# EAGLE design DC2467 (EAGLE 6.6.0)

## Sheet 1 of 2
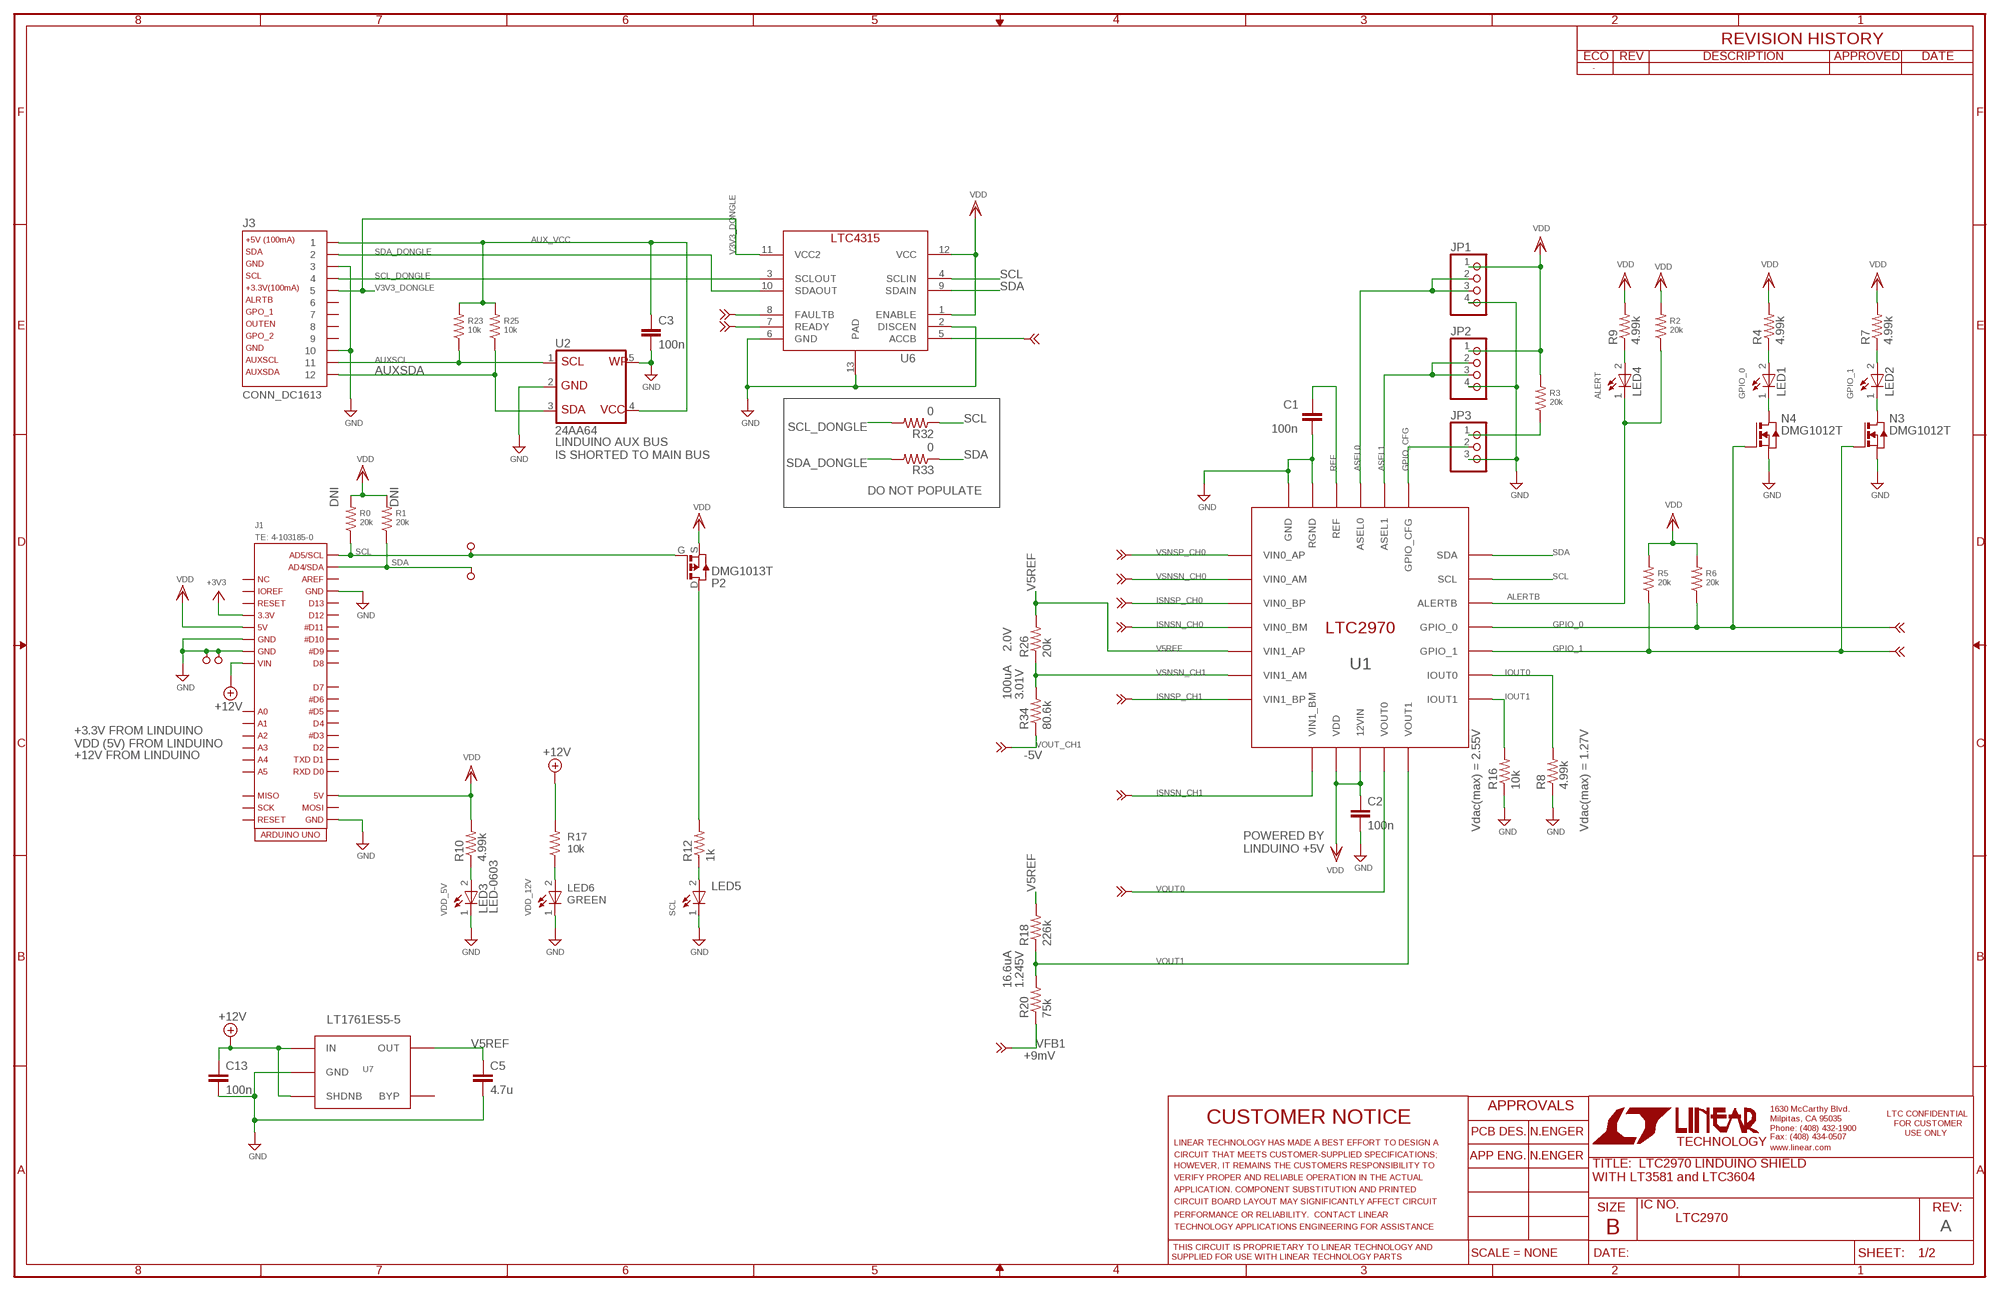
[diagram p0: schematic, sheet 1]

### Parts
C1  100n  CC0603_BOX  [C0603_BOX]
C2  100n  CC0603_BOX  [C0603_BOX]
C3  100n  CC0603_BOX  [C0603_BOX]
C5  4.7u  CC0603_BOX  [C0603_BOX]
C13  100n  CC0603_BOX  [C0603_BOX]
J1  TE: 4-103185-0  ARDUINO_UNO_MINI_SHIELD_SPIFL  [ADRUINO_UNO_STD_SHIELD_SPI]
J3  CONN_DC1613  [CONN_DC1613]
JP1  PINHD-1X4  [1X04]
JP2  PINHD-1X4  [1X04]
JP3  PINHD-1X3  [1X03]
LED1  LED-0603  [CHIPLED_0603]
LED2  LED-0603  [CHIPLED_0603]
LED3  LED-0603  [CHIPLED_0603]
LED4  LED-0603  [CHIPLED_0603]
LED5  LED-0603  [CHIPLED_0603]
LED6  GREEN  LED-0603  [CHIPLED_0603]
N3  DMG1012T  [SOT523-3]
N4  DMG1012T  [SOT523-3]
P2  DMG1013T  [SOT523-3]
R0  20k  RR0603_BOX  [R0603_BOX]
R1  20k  RR0603_BOX  [R0603_BOX]
R2  20k  RR0603_BOX  [R0603_BOX]
R3  20k  RR0603_BOX  [R0603_BOX]
R4  4.99k  RR0603_BOX  [R0603_BOX]
R5  20k  RR0603_BOX  [R0603_BOX]
R6  20k  RR0603_BOX  [R0603_BOX]
R7  4.99k  RR0603_BOX  [R0603_BOX]
R8  4.99k  RR0603_BOX  [R0603_BOX]
R9  4.99k  RR0603_BOX  [R0603_BOX]
R10  4.99k  RR0603_BOX  [R0603_BOX]
R12  1k  RR0603_BOX  [R0603_BOX]
R16  10k  RR0603_BOX  [R0603_BOX]
R17  10k  RR0603_BOX  [R0603_BOX]
R18  226k  RR0603_BOX  [R0603_BOX]
R20  75k  RR0603_BOX  [R0603_BOX]
R23  10k  RR0603_BOX  [R0603_BOX]
R25  10k  RR0603_BOX  [R0603_BOX]
R26  20k  RR0603_BOX  [R0603_BOX]
R32  0  RR0603_BOX  [R0603_BOX]
R33  0  RR0603_BOX  [R0603_BOX]
R34  80.6k  RR0603_BOX  [R0603_BOX]
TP1  TESPOINT_SMDSMD  [TESPOINT_SMD]
TP3  TESPOINT_SMDSMD  [TESPOINT_SMD]
TP4  TESTPOINT_BIG  [TP1]
TP5  TURRET_SMALL_2308TP  [TURRET_SMALL_2308]
TP6  TURRET_SMALL_2308TP  [TURRET_SMALL_2308]
TP7  TURRET_SMALL_2308TP  [TURRET_SMALL_2308]
TP10  TESPOINT_SMDSMD  [TESPOINT_SMD]
U1  LTC2970  [QFN-24]
U2  24AA64  [SOT-23-5]
U6  LTC4315  [DFN-12]
U7  LT1761ES5-5  [TSOT23-5]
U$1  FRAME_DC2467  [FRAME_DC2467]

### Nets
+3V3: J1.3V3
+12V: C13.1 J1.VIN R17.2 U7.P$1(IN) U7.P$3(SHDNB) ; also sheet 2
ALERTB: LED4.C R2.1 U1.P$17(ALERTB)
ASEL0: JP1.2 JP1.3 U1.P$22(ASEL0)
ASEL1: JP2.2 JP2.3 U1.P$21(ASEL1)
AUX_VCC: C3.1 J3.1 R23.2 R25.2 U2.4
AUXSCL: J3.11 R23.1 U2.1
AUXSDA: J3.12 R25.1 U2.3
GND: C1.2 C2.2 C3.2 C5.2 C13.2 J1.GND1 J1.GND2 J1.GND3 J1.GND4 J3.3 J3.10 JP1.4 JP2.4 JP3.3 LED3.C LED5.C LED6.C N3.S N4.S R8.1 R16.1 TP4.TP TP5.TP1 U1.P$24(RGND) U1.P$25(GND) U2.2 U2.5 U6.2(DISCEN) U6.6(GND) U6.13(PAD) U7.P$2(GND) ; also sheet 2
GPIO_0: N4.G R6.1 U1.P$16(GPIO_0) ; also sheet 2
GPIO_1: N3.G R5.1 U1.P$15(GPIO_1) ; also sheet 2
GPIO_CFG: JP3.2 U1.P$20(GPIO_CFG)
IOUT0: R8.2 U1.P$14(IOUT0)
IOUT1: R16.2 U1.P$13(IOUT1)
ISNSN_CH0: U1.P$4(VIN0_BM) ; also sheet 2
ISNSN_CH1: U1.P$8(VIN1_BM) ; also sheet 2
ISNSP_CH0: U1.P$3(VIN0_BP) ; also sheet 2
ISNSP_CH1: U1.P$7(VIN1_BP) ; also sheet 2
N$1: LED1.C N4.D
N$2: LED1.A R4.1
N$3: LED2.C N3.D
N$4: LED2.A R7.1
N$6: LED3.A R10.1
N$7: LED4.A R9.1
N$9: LED5.A R12.1
N$10: P2.D R12.2
N$11: LED6.A R17.1
N$16: JP3.1 R3.1
N$26: TP3.P$1 U6.8(FAULTB)
N$29: TP10.P$1 U6.7(READY)
N$30: TP1.P$1 U6.5(ACCB)
REF: C1.1 U1.P$23(REF)
SCL: J1.SCL P2.G R0.1 R32.1 TP7.TP1 U1.P$18(SCL) U6.4(SCLIN)
SCL_DONGLE: J3.4 R32.2 U6.3(SCLOUT)
SDA: J1.SDA R1.1 R33.1 TP6.TP1 U1.P$19(SDA) U6.9(SDAIN)
SDA_DONGLE: J3.2 R33.2 U6.10(SDAOUT)
V3V3_DONGLE: J3.5 U6.11(VCC2)
V5REF: C5.1 R18.2 R26.2 U1.P$5(VIN1_AP) U7.P$5(OUT)
VDD: C2.1 J1.5V J1.5V1 JP1.1 JP2.1 P2.S R0.2 R1.2 R2.2 R3.2 R4.2 R5.2 R6.2 R7.2 R9.2 R10.2 U1.P$9(VDD) U1.P$10(12VIN) U6.1(ENABLE) U6.12(VCC)
VFB1: R20.1 ; also sheet 2
VOUT0: U1.P$11(VOUT0) ; also sheet 2
VOUT1: R18.1 R20.2 U1.P$12(VOUT1)
VOUT_CH1: R34.1 ; also sheet 2
VSNSN_CH0: U1.P$2(VIN0_AM) ; also sheet 2
VSNSN_CH1: R26.1 R34.2 U1.P$6(VIN1_AM)
VSNSP_CH0: U1.P$1(VIN0_AP) ; also sheet 2
Unconnected: J1.A0 J1.A1 J1.A2 J1.A3 J1.A4 J1.A5 J1.D0 J1.D1 J1.D2 J1.D3 J1.D4 J1.D5 J1.D6 J1.D7 J1.D8 J1.D9 J1.D10 J1.D11 J1.D12 J1.D13 J1.MISO J1.MOSI J1.NC J1.REF J1.RST1 J1.RST2 J1.SCK J1.VIO J3.6 J3.7 J3.8 J3.9 U7.P$4(BYP)

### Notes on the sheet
- ALERT | GPIO_0 | GPIO_1
- LINDUINO AUX BUS 
  IS SHORTED TO MAIN BUS
- DO NOT POPULATE
- DNI | DNI
- 2.0V
- 100uA | 3.01V
- +3.3V FROM LINDUINO
  VDD (5V) FROM LINDUINO
- +12V FROM LINDUINO | -5V
- POWERED BY
  LINDUINO +5V
- Vdac(max) = 2.55V | Vdac(max) = 1.27V
- VDD_5V | VDD_12V | SCL
- 16.6uA | 1.245V
- LT1761ES5-5
- +9mV
- A

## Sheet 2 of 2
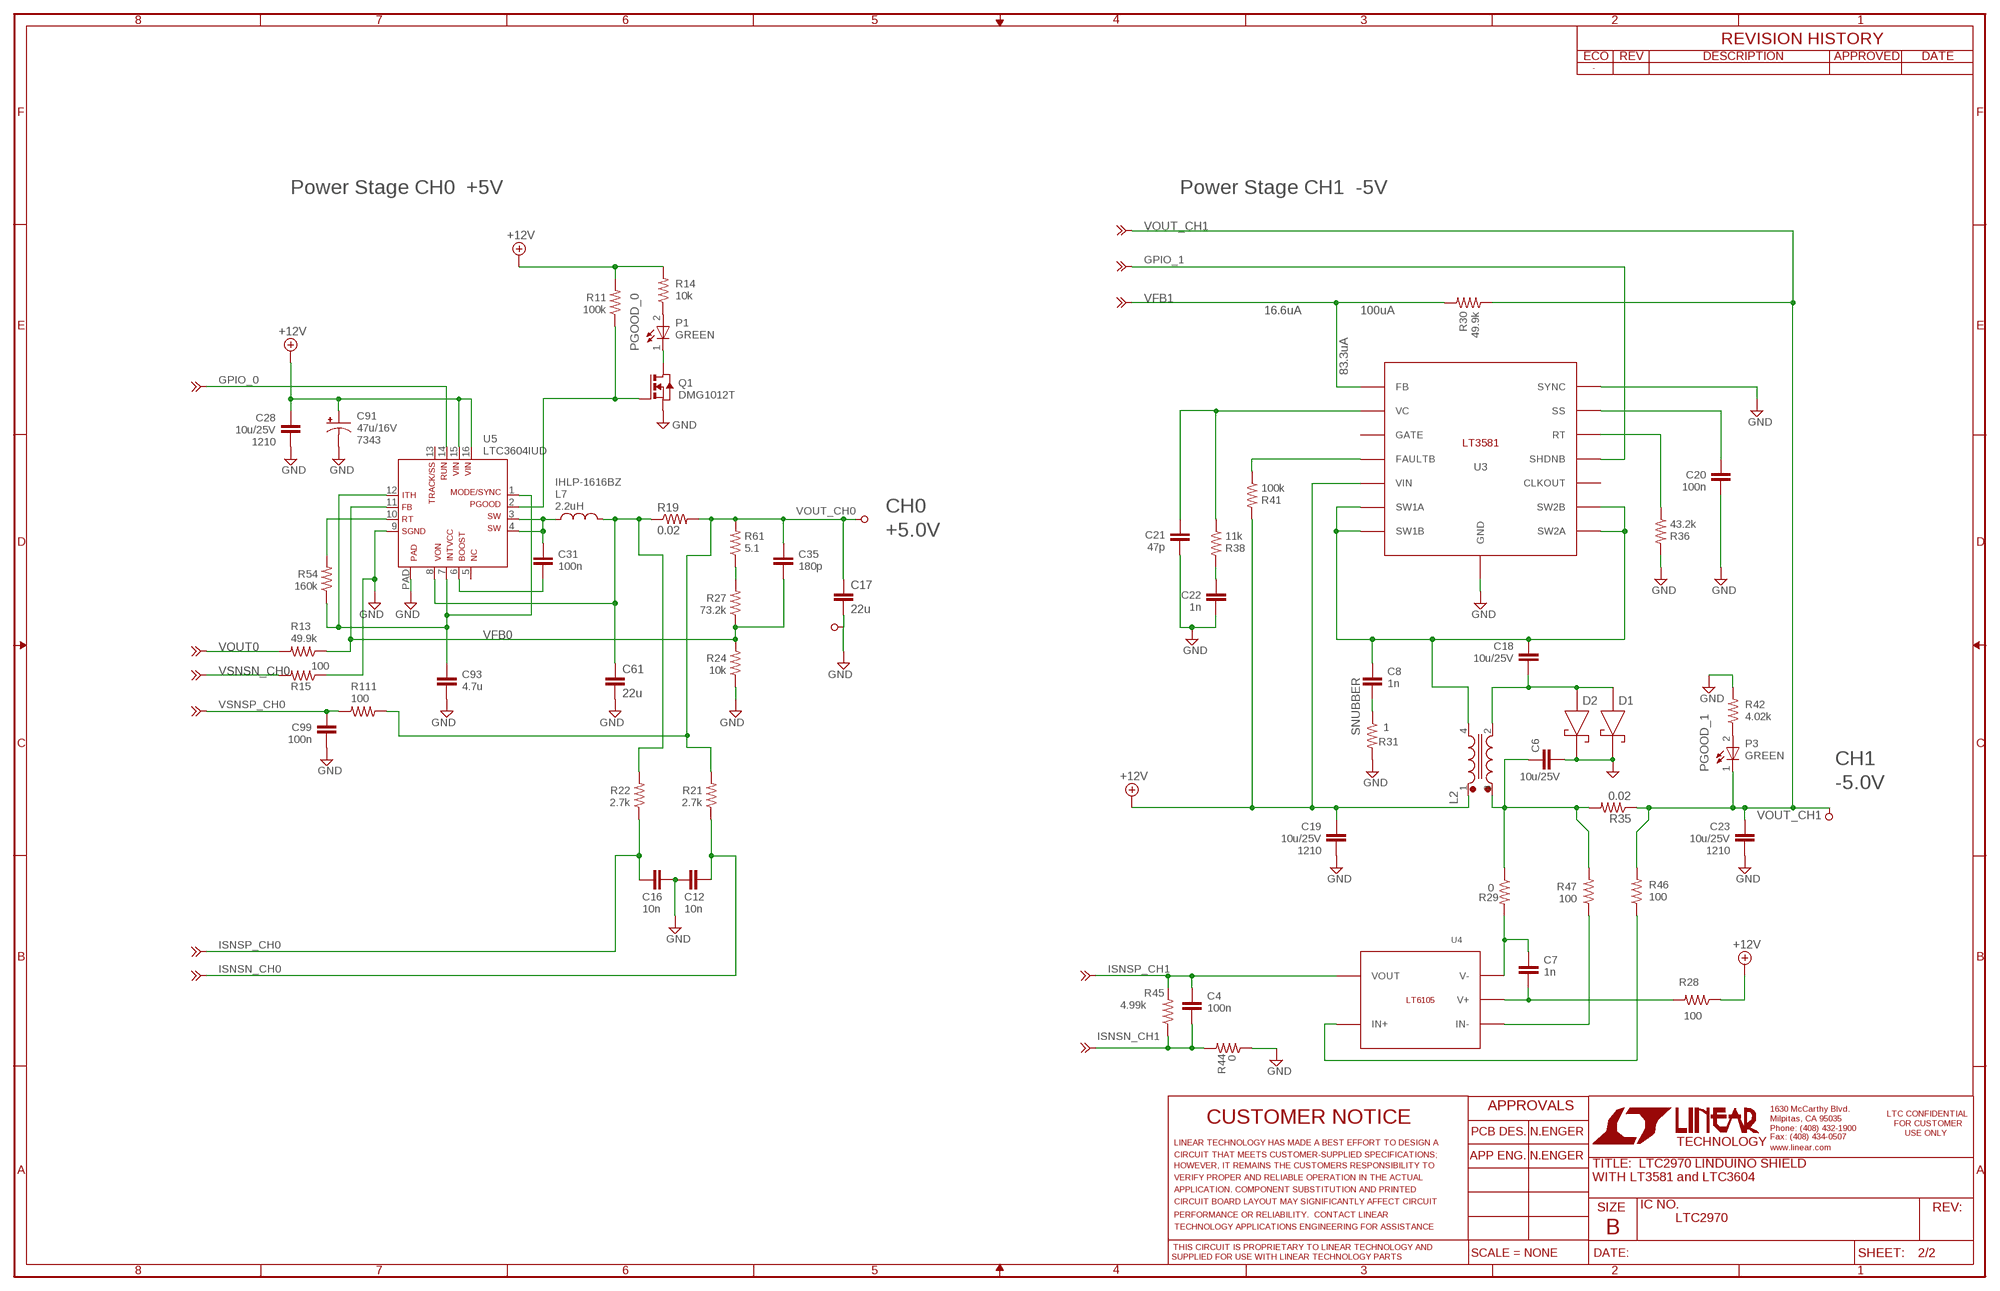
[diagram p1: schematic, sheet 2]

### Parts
C4  100n  CC0603_BOX  [C0603_BOX]
C6  10u/25V  CC1210_BOX  [C1210_BOX]
C7  1n  CC0603_BOX  [C0603_BOX]
C8  1n  CC0603_BOX  [C0603_BOX]
C12  10n  CC0603_BOX  [C0603_BOX]
C16  10n  CC0603_BOX  [C0603_BOX]
C17  22u  CC1210_BOX  [C1210_BOX]
C18  10u/25V  CC1210_BOX  [C1210_BOX]
C19  10u/25V  CC1210_BOX  [C1210_BOX]
C20  100n  CC0603_BOX  [C0603_BOX]
C21  47p  CC0603_BOX  [C0603_BOX]
C22  1n  CC0603_BOX  [C0603_BOX]
C23  10u/25V  CC1210_BOX  [C1210_BOX]
C28  10u/25V  CC1210_BOX  [C1210_BOX]
C31  100n  CC0603_BOX  [C0603_BOX]
C35  180p  CC0603_BOX  [C0603_BOX]
C61  22u  CC1210_BOX  [C1210_BOX]
C91  47u/16V  CPOL-USCT7343  [CT7343]
C93  4.7u  CC0603_BOX  [C0603_BOX]
C99  100n  CC0603_BOX  [C0603_BOX]
D1  DFLS220L  [POWERDI-123]
D2  DFLS220L  [POWERDI-123]
L2  WE-TDC_8038  [WE-TDC_80XX]
L7  2.2uH  LVISHAY-IHLP1616AB  [IHLP_1616AB]
P1  GREEN  LED-0603  [CHIPLED_0603]
P3  GREEN  LED-0603  [CHIPLED_0603]
Q1  DMG1012T  [SOT523-3]
R11  100k  RR0603_BOX  [R0603_BOX]
R13  49.9k  RR0603_BOX  [R0603_BOX]
R14  10k  RR0603_BOX  [R0603_BOX]
R15  100  RR0603_BOX  [R0603_BOX]
R19  0.02  RR1210  [R1210]
R21  2.7k  RR0603_BOX  [R0603_BOX]
R22  2.7k  RR0603_BOX  [R0603_BOX]
R24  10k  RR0603_BOX  [R0603_BOX]
R27  73.2k  RR0603_BOX  [R0603_BOX]
R28  100  RR0603_BOX  [R0603_BOX]
R29  0  RR0603_BOX  [R0603_BOX]
R30  49.9k  RR0603_BOX  [R0603_BOX]
R31  1  RR0603_BOX  [R0603_BOX]
R35  0.02  RR1210  [R1210]
R36  43.2k  RR0603_BOX  [R0603_BOX]
R38  11k  RR0603_BOX  [R0603_BOX]
R41  100k  RR0603_BOX  [R0603_BOX]
R42  4.02k  RR0603_BOX  [R0603_BOX]
R44  0  RR0603_BOX  [R0603_BOX]
R45  4.99k  RR0603_BOX  [R0603_BOX]
R46  100  RR0603_BOX  [R0603_BOX]
R47  100  RR0603_BOX  [R0603_BOX]
R54  160k  RR0603_BOX  [R0603_BOX]
R61  5.1  RR0603_BOX  [R0603_BOX]
R111  100  RR0603_BOX  [R0603_BOX]
TP2  TESTPOINT_BIG  [TP1]
TP8  TESTPOINT_BIG  [TP1]
TP9  TESTPOINT_BIG  [TP1]
U3  LT3581  [DFN-14]
U4  LT6105  [DFN-6]
U5  LTC3604IUD  [QFN16_3X3]
U$3  FRAME_DC2467  [FRAME_DC2467]
VSNSN1  TESPOINT_SMD  TESPOINT_SMDVIA  [VIA]
VSNSN2  TESPOINT_SMD  TESPOINT_SMDVIA  [VIA]
VSNSN3  TESPOINT_SMD  TESPOINT_SMDVIA  [VIA]
VSNSN4  TESPOINT_SMD  TESPOINT_SMDVIA  [VIA]
VSNSN11  TESPOINT_SMD  TESPOINT_SMDVIA  [VIA]
VSNSN56  TESPOINT_SMD  TESPOINT_SMDVIA  [VIA]
VSNSN57  TESPOINT_SMD  TESPOINT_SMDVIA  [VIA]
VSNSN58  TESPOINT_SMD  TESPOINT_SMDVIA  [VIA]
VSNSN59  TESPOINT_SMD  TESPOINT_SMDVIA  [VIA]

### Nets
+12V: C19.2 C28.2 C91.+ L2.1 R11.2 R14.2 R28.1 R41.2 U3.P$5(VIN) U5.15 U5.16 ; also sheet 1
GND: C6.1 C12.2 C16.1 C17.2 C19.1 C20.1 C21.1 C22.1 C23.1 C28.1 C61.2 C91.- C93.2 C99.1 D1.P$1 D2.P$1 Q1.S R15.1 R24.1 R31.2 R36.2 R42.2 R44.1 TP9.TP U3.P$14(SYNC) U3.P$15(GND) U5.9 U5.PAD ; also sheet 1
GPIO_0: U5.14 VSNSN11.1 ; also sheet 1
GPIO_1: U3.P$11(SHDNB) VSNSN2.1 ; also sheet 1
INTVCC_LTC3604: C93.1 R54.1 U5.1 U5.7 U5.12
ISNSN_CH0: C12.1 R21.1 VSNSN56.1 ; also sheet 1
ISNSN_CH1: C4.1 R44.2 R45.1 ; also sheet 1
ISNSP_CH0: C16.2 R22.1 VSNSN57.1 ; also sheet 1
ISNSP_CH1: C4.2 R45.2 U4.P$4(VOUT) VSNSN4.1 ; also sheet 1
N$5: R47.1 U4.P$1(IN-)
N$8: R27.2 R61.1
N$12: C7.2 R29.2 U4.P$3(V-) U4.P$9(V-)
N$13: C7.1 R28.2 U4.P$2(V+)
N$14: C8.1 R31.1
N$15: C18.1 D1.P$2 D2.P$2 L2.2
N$18: C8.2 C18.2 L2.4 U3.P$6(SW1A) U3.P$7(SW1B) U3.P$8(SW2A) U3.P$9(SW2B)
N$19: P1.A R14.1
N$20: P1.C Q1.D
N$21: R41.1 U3.P$4(FAULTB)
N$22: R36.1 U3.P$12(RT)
N$23: C20.2 U3.P$13(SS)
N$25: Q1.G R11.1 U5.2
N$27: C6.2 L2.3 R29.1 R35.2 R47.2
N$28: P3.A R42.1
N$31: C22.2 R38.2
N$32: C21.2 R38.1 U3.P$2(VC)
N$33: R46.1 U4.P$6(IN+)
N$70: C31.2 U5.6
N$78: R54.2 U5.10
SW1: C31.1 L7.1 U5.3 U5.4
V1: C61.1 L7.2 R19.1 R22.2 U5.8
VFB0: C35.2 R13.1 R24.2 R27.1 U5.11
VFB1: R30.2 U3.P$1(FB) VSNSN3.1 ; also sheet 1
VOUT0: R13.2 VSNSN58.1 ; also sheet 1
VOUT_CH0: C17.1 C35.1 R19.2 R21.2 R61.2 R111.1 TP8.TP
VOUT_CH1: C23.2 P3.C R30.1 R35.1 R46.2 TP2.TP ; also sheet 1
VSNSN_CH0: R15.2 VSNSN1.1 ; also sheet 1
VSNSP_CH0: C99.2 R111.2 VSNSN59.1 ; also sheet 1
Unconnected: U3.P$3(GATE) U3.P$10(CLKOUT) U5.5 U5.13

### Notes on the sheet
- Power Stage CH0  +5V | Power Stage CH1  -5V
- 16.6uA | 100uA
- PGOOD_0
- 83.3uA
- 1210
- 7343
- IHLP-1616BZ
- CH0
- +5.0V
- SNUBBER
- CH1
- PGOOD_1
- -5.0V
- 1210 | 1210

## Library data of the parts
C1-C8 C12 C13 C16-C23 C28 C31 C35 C61 C93 C99 = kalin:C: CAPACITOR, European symbol
C91 = rcl:CPOL-US: POLARIZED CAPACITOR, American symbol
D1 D2 = nengerLib:DFLS220L: DIODES INC DFLS220L
J1 = FOO:ARDUINO_UNO_MINI_SHIELD_SPI: Arduino UNO Mini Shield With SPI
J3 = kalin:CONN_DC1613: Connector for LT DC1613 USB Dongle
JP1 JP2 = LIBSnengerLib:PINHD-1X4: PIN HEADER
JP3 = LIBSnengerLib:PINHD-1X3: PIN HEADER
L2 = Wurth_Elektronik_Passive_rev15f:WE-TDC: SEPIC SMD Coupled Inductor Characteristics Core material: NiZn Low profile Magnetical shielded which results in a low leakage field 8x8 mm case 1:1 transformer Low self-losses High self resonance frequency Coupled inductor with two identical windings Operating temperature: –40 °C up to +125 °C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
L7 = kalin:L: Inductor
LED1-LED6 P1 P3 = kalin:LED-0603: SMD LED in R0603
N3 N4 Q1 = nengerLib:DMG1012T: Diodes Inc. N-Channel Enhancement Mode N-MOSFET
P2 = FOO:DMG1013T: Diodes Inc. P-Channel Enhancement Mode P-MOSFET
R0 R1-R36 R38 R41 R42 R44-R47 R54 R61 R111 = kalin:R: RESISTOR, American symbol
TP1 TP3 TP10 VSNSN1-VSNSN4 VSNSN11 VSNSN56-VSNSN59 = kalin:TESPOINT_SMD: SMALL SMD Test Point
TP2 TP4 TP8 TP9 = kalin:TESTPOINT_BIG: Large Test Point
TP5-TP7 = kalin:TURRET_SMALL_2308: Small Test Turret Mill-Max 2308
U1 = LTC-DEVICES:LTC2970: LTC2970 Dual I2C Power Supply Monitor and Margining Controller
U2 = kalin:24AA64: 64K I2C? Serial EEPROM
U3 = LTC-DEVICES:LT3581: LT3581 3.3A Boost/Inverting DC/DC Converter with Fault Protection
U4 = LTC-DEVICES:LT6105
U5 = kalin:LTC3604: 2.5A, 15V Monolithic Synchronous Step-Down Regulator
U6 = LTC-DEVICES:LTC4315: 2-Wire Bus Buffer with High Noise Margin
U7 = nengerLib:LT1761ES5-5
U$1 U$3 = nengerFramesLib:FRAME_DC2467

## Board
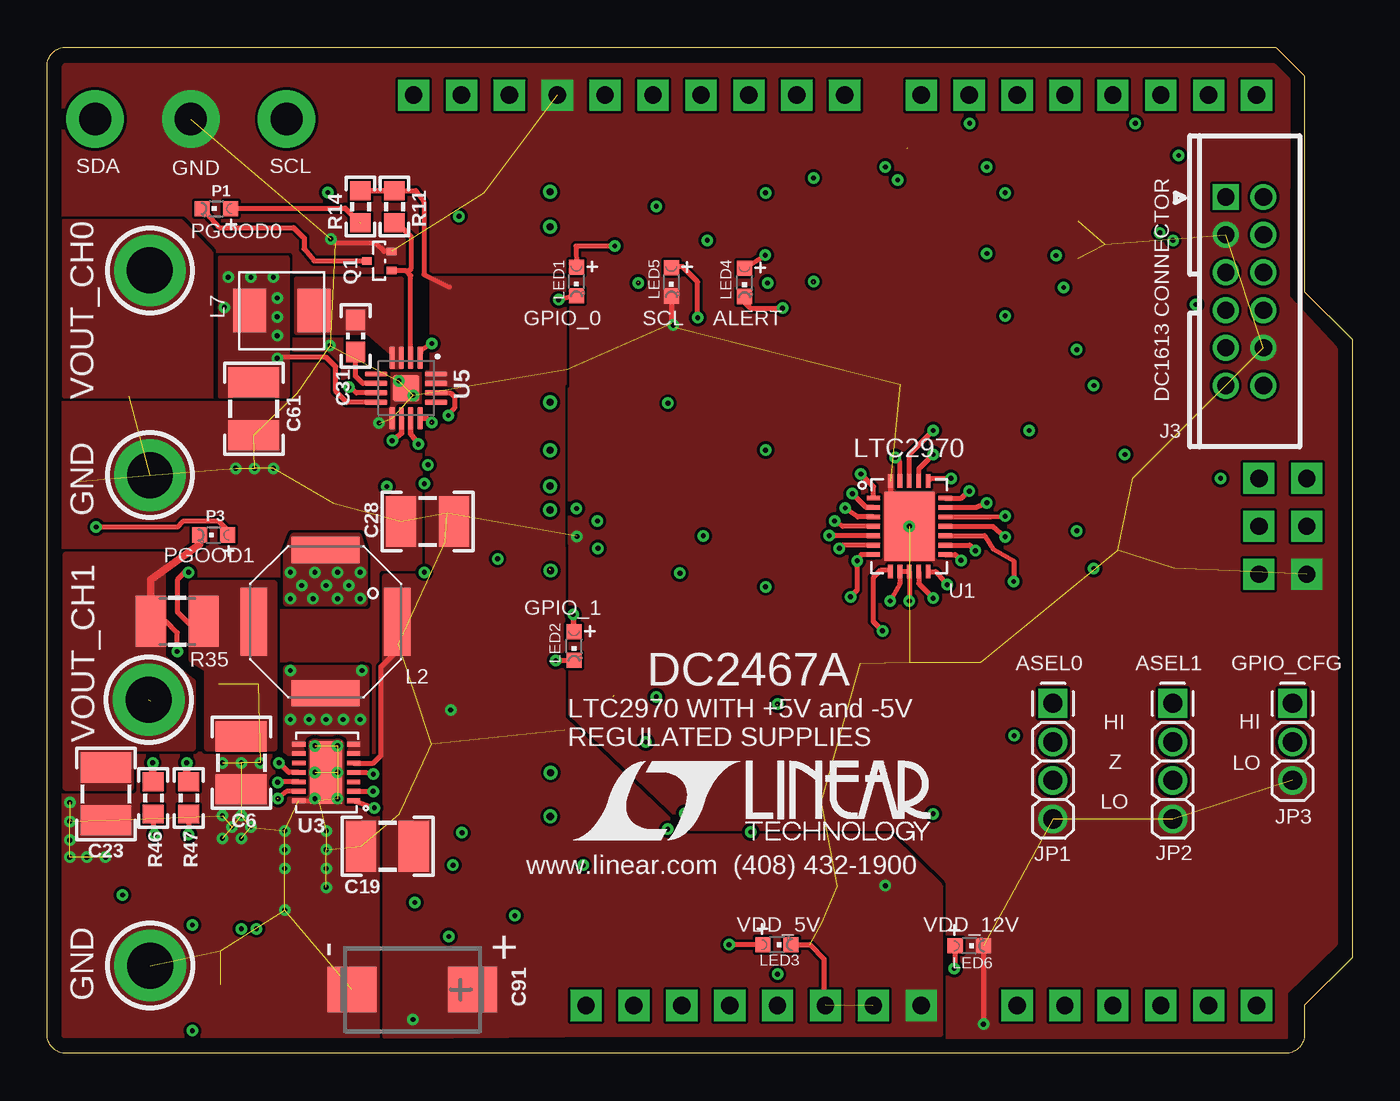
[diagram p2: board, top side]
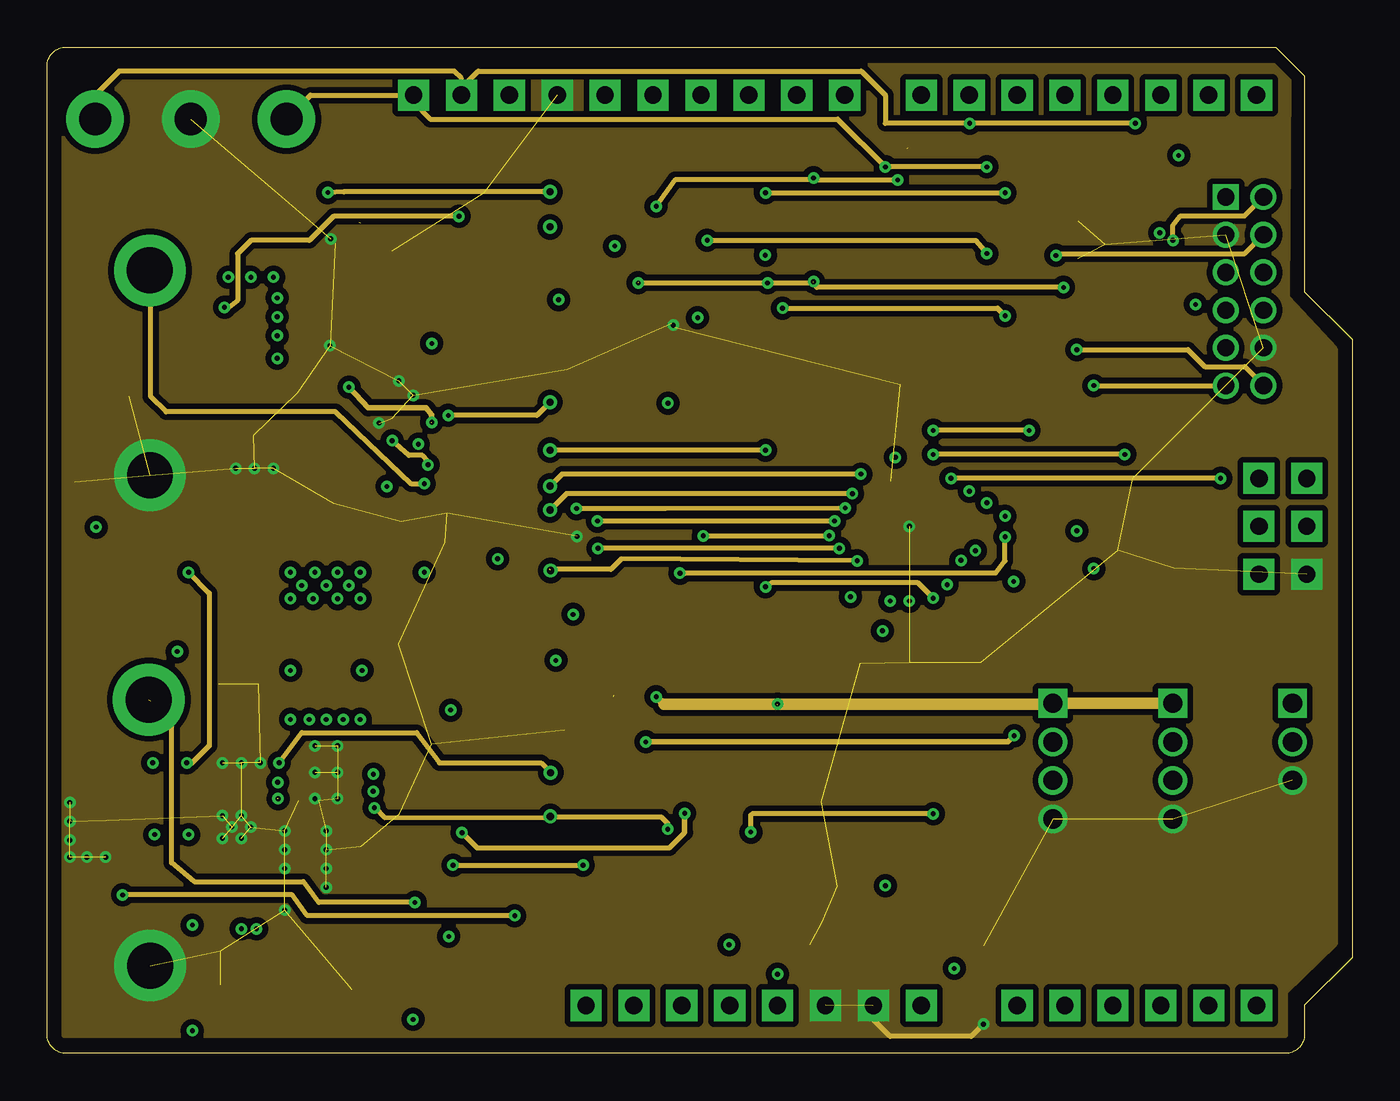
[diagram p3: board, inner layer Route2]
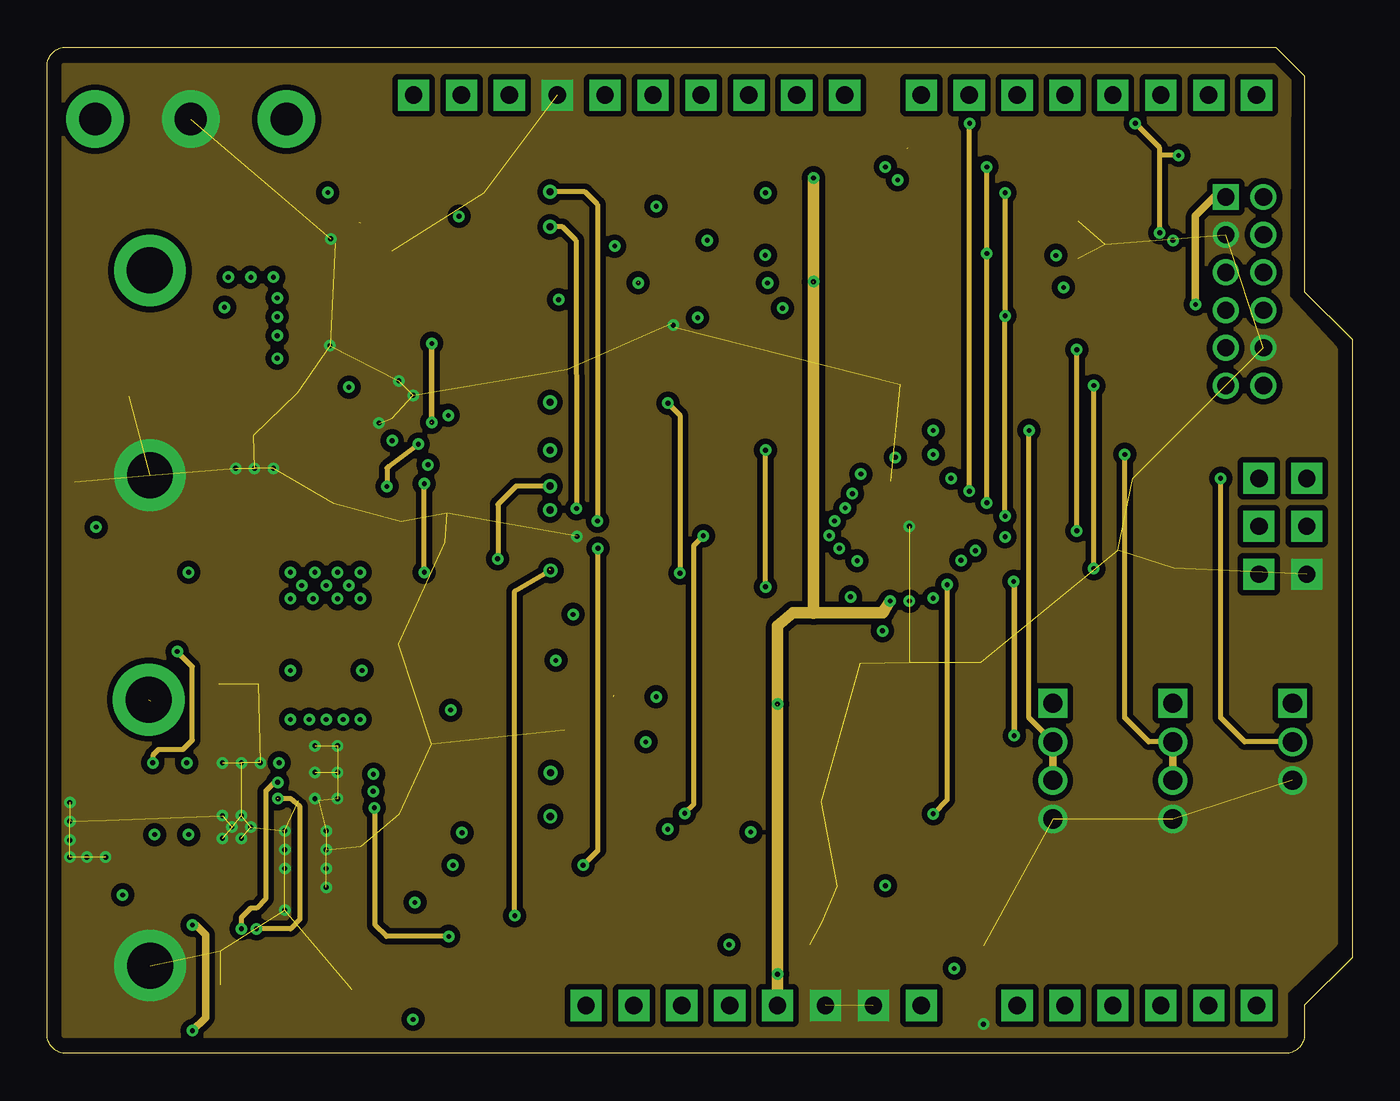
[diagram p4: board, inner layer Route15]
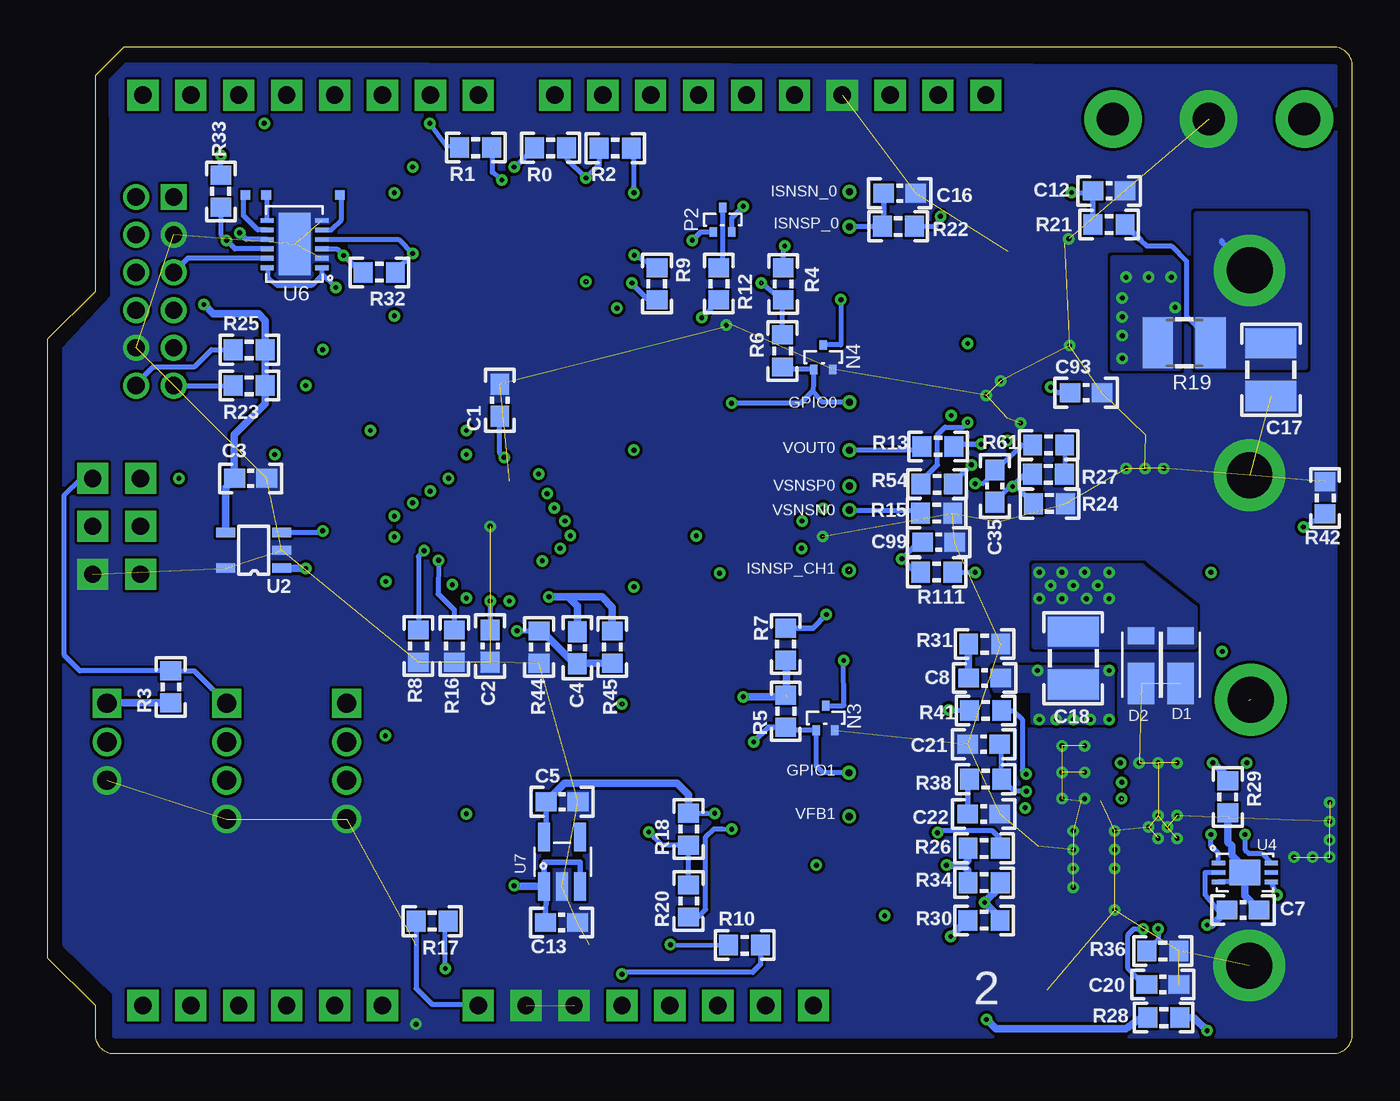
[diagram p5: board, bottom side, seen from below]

Size 69.22 x 53.34 mm. Coordinates in mm from the lower left corner, seen from the top.
Copper layers (1+2*15+16): Top 0.07mm / dielectric 0.23mm / Route2 0.035mm / dielectric 1.01mm / Route15 0.035mm / dielectric 0.2mm / Bottom 0.07mm
Design rules "nicks-panel": minimum track width 6mil, minimum drill 10mil, track to track 6mil, track to pad 6mil, pad to pad 6mil, via to via 6mil, smd to smd 6mil, copper to edge 20mil, drill to drill 8mil, minimum pad ring 7mil, minimum via ring 7mil, stop-mask expansion 2.5mil, vias tented up to drill 14mil, thermal gap 10mil

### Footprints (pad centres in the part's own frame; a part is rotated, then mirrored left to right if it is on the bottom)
C0603_BOX = smd 1.1 x 1: 1 -0.85,0; 2 0.85,0
C1210_BOX = smd 1.6 x 2.7: 1 -1.4,0; 2 1.4,0
CT7343 = smd 2.6 x 2.4: + -3.2,0; - 3.2,0
POWERDI-123 = smd 2.2 x 1.4: P$1 -1.6,0 | smd 0.9 x 1.4: P$2 0.95,0
ADRUINO_UNO_STD_SHIELD_SPI = drill 0.914 pad 1.651 square: 3V3 18.415,2.54; 5V 20.955,2.54; 5V1 49.022,30.48; A0 33.655,2.54; A1 36.195,2.54; A2 38.735,2.54; A3 41.275,2.54; A4 43.815,2.54; A5 46.355,2.54; D0 46.355,50.8; D1 43.815,50.8; D2 41.275,50.8; D3 38.735,50.8; D4 36.195,50.8; D5 33.655,50.8; D6 31.115,50.8; D7 28.575,50.8; D8 24.511,50.8; D9 21.971,50.8; D10 19.431,50.8; D11 16.891,50.8; D12 14.351,50.8; D13 11.811,50.8; GND1 23.495,2.54; GND2 26.035,2.54; GND3 9.271,50.8; GND4 49.022,25.4; MISO 46.482,30.48; MOSI 49.022,27.94; NC 10.795,2.54; REF 6.731,50.8; RST1 15.875,2.54; RST2 46.482,25.4; SCK 46.482,27.94; SCL 1.651,50.8; SDA 4.191,50.8; VIN 28.575,2.54; VIO 13.335,2.54
CONN_DC1613 = drill 0.914 square: 1 -5,-1 | drill 0.914: 2 -5,1; 3 -3,-1; 4 -3,1; 5 -1,-1; 6 -1,1; 7 1,-1; 8 1,1; 9 3,-1; 10 3,1; 11 5,-1; 12 5,1
1X04 = drill 1.016 square: 1 -2.05,0 | drill 1.016: 2 0,0; 3 2.04,0; 4 4.09,0
1X03 = drill 1.016 square: 1 -2.05,0 | drill 1.016: 2 0,0; 3 2.04,0
WE-TDC_80XX = smd 3.6 x 1.4: 1 0,3.8; 3 0,-3.8 | smd 1.4 x 3.6: 2 -3.8,0; 4 3.8,0
IHLP_1616AB = smd 1.75 x 2.3: 1 -1.7,0; 2 1.7,0
CHIPLED_0603 = smd 0.8 x 0.8: A 0,-0.75; C 0,0.75
SOT523-3 = smd 0.4 x 0.51: D 0,0.65; G -0.5,-0.65; S 0.5,-0.65
R0603_BOX = smd 1 x 1.1: 1 -0.85,0; 2 0.85,0
R1210 = smd 1.6 x 2.7: 1 -1.4,0; 2 1.4,0
TESPOINT_SMD = smd 0.508 x 0.508: P$1 0,0
TP1 = drill 2.438 pad 3.81: TP 0,0
TURRET_SMALL_2308 = drill 1.702 pad 3.048: TP1 0,0
QFN-24 = smd 0.7 x 0.25: P$1 -1.9,1.5; P$2 -1.9,1; P$3 -1.9,0.5; P$4 -1.9,0; P$5 -1.9,-0.5; P$6 -1.9,-1; P$7 -1.9,-1.5; P$13 1.9,-1.5; P$14 1.9,-1; P$15 1.9,-0.5; P$16 1.9,0; P$17 1.9,0.5; P$18 1.9,1; P$19 1.9,1.5 | smd 0.25 x 0.7: P$8 -1,-2.4; P$9 -0.5,-2.4; P$10 0,-2.4; P$11 0.5,-2.4; P$12 1,-2.4; P$20 1,2.4; P$21 0.5,2.4; P$22 0,2.4; P$23 -0.5,2.4; P$24 -1,2.4 | smd 2.65 x 3.65: P$25 0,0
SOT-23-5 = smd 1 x 0.5: 1 -1.649,0.95; 2 -1.649,0; 3 -1.649,-0.95; 4 1.333,-0.95; 5 1.333,0.95
DFN-14 = smd 0.25 x 0.7: P$1 -1.5,-1.45; P$2 -1,-1.45; P$3 -0.5,-1.45; P$4 0,-1.45; P$5 0.5,-1.45; P$6 1,-1.45; P$7 1.5,-1.45; P$8 1.5,1.45; P$9 1,1.45; P$10 0.5,1.45; P$11 0,1.45; P$12 -0.5,1.45; P$13 -1,1.45; P$14 -1.5,1.45 | smd 3.3 x 1.7: P$15 0,0
DFN-6 = smd 0.25 x 0.7: P$1 -0.5,-1.4; P$2 0,-1.4; P$3 0.5,-1.4; P$4 0.5,1.4; P$5 0,1.4; P$6 -0.5,1.4 | smd 1.35 x 1.65: P$9 0,0
QFN16_3X3 = smd 1.2 x 0.3: 1 -1.711,0.734; 2 -1.711,0.234; 3 -1.711,-0.266; 4 -1.711,-0.766; 9 1.489,-0.766; 10 1.489,-0.266; 11 1.489,0.234; 12 1.489,0.734 | smd 0.3 x 1.2: 5 -0.861,-1.616; 6 -0.361,-1.616; 7 0.139,-1.616; 8 0.639,-1.616; 13 0.639,1.584; 14 0.139,1.584; 15 -0.361,1.584; 16 -0.861,1.584 | smd 1.4 x 1.4: PAD -0.111,-0.016
DFN-12 = smd 0.7 x 0.25: 1 -1.45,1.25; 2 -1.45,0.75; 3 -1.45,0.25; 4 -1.45,-0.25; 5 -1.45,-0.75; 6 -1.45,-1.25; 7 1.45,-1.25; 8 1.45,-0.75; 9 1.45,-0.25; 10 1.45,0.25; 11 1.45,0.75; 12 1.45,1.25 | smd 1.7 x 3.3: 13 0,0
TSOT23-5 = smd 0.63 x 1.5: P$1 -0.95,-1.31; P$2 0,-1.31; P$3 0.95,-1.31; P$4 0.95,1.31; P$5 -0.95,1.31
VIA = drill 0.381: 1 0,0

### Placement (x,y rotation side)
C1  45.21,34.62 90 bottom
C2  45.72,21.59 270 bottom
C3  58.42,30.48 0 bottom
C4  41.1,21.5 90 bottom
C5  41.91,13.34 0 bottom
C6  10.3,15.4 90 top
C7  5.8,7.6 0 bottom
C8  19.5,19.9 0 bottom
C12  12.9,45.72 0 bottom
C13  41.94,6.93 0 bottom
C16  24,45.59 180 bottom
C17  4.32,36.25 270 bottom
C18  14.8,20.95 270 bottom
C19  18.05,10.98 0 top
C20  10.05,3.65 180 bottom
C21  19.55,16.39 0 bottom
C22  19.55,12.69 180 bottom
C23  3.12,13.75 90 top
C28  20.18,28.19 0 top
C31  16.36,38.02 270 top
C35  18.96,30.07 270 bottom
C61  10.96,34.17 270 top
C91  19.37,3.38 180 top
C93  14.12,35.03 0 bottom
C99  21.94,27.1 180 bottom
D1  9.1,21.2 90 bottom
D2  11.2,21.2 90 bottom
DRILEGEND  [DRILEGEND]  not placed on the board
J1  17.78,0 0 top
J3  63.5,40.4 270 top
JP1  53.34,16.51 270 top
JP2  59.69,16.51 270 top
JP3  66.04,16.51 270 top
L2  14.77,22.89 270 top
L7  12.45,39.37 180 top
LED1  28.07,40.92 180 top
LED2  27.94,21.59 180 top
LED3  38.7,5.76 270 top
LED4  36.98,40.87 180 top
LED5  33.1,40.9 180 top
LED6  48.9,5.7 270 top
N3  27.94,17.78 0 bottom
N4  28.07,36.91 0 bottom
P1  8.98,44.78 90 top
P2  33.4,44.2 0 bottom
P3  8.83,27.48 90 top
Q1  17.61,42.01 90 top
R0  42.52,48.01 0 bottom
R1  46.49,48.02 0 bottom
R2  39.09,47.98 180 bottom
R3  62.66,19.43 90 bottom
R4  30.18,40.79 270 bottom
R5  30.05,18.14 90 bottom
R6  30.23,37.24 90 bottom
R7  30.05,21.69 270 bottom
R8  49.53,21.59 90 bottom
R9  36.88,40.8 270 bottom
R10  32.23,5.74 0 bottom
R11  18.42,44.88 90 top
R12  33.6,40.8 90 bottom
R13  21.97,32.17 180 bottom
R14  16.61,44.88 90 top
R15  22.05,28.63 180 bottom
R16  47.62,21.59 90 bottom
R17  48.8,7 180 bottom
R18  35.2,11.89 90 bottom
R19  8.92,37.67 0 bottom
R20  35.2,8.08 90 bottom
R21  12.9,43.94 0 bottom
R22  24.08,43.84 0 bottom
R23  58.5,35.4 0 bottom
R24  16.06,29.14 180 bottom
R25  58.5,37.3 0 bottom
R26  19.52,10.87 0 bottom
R27  16.12,30.71 0 bottom
R28  10,1.9 0 bottom
R29  6.6,13.6 270 bottom
R30  19.53,7.05 180 bottom
R31  19.5,21.7 0 bottom
R32  51.6,41.4 180 bottom
R33  60,45.7 270 bottom
R34  19.52,9.04 180 bottom
R35  6.9,22.9 0 top
R36  10.05,5.43 0 bottom
R38  19.45,14.53 180 bottom
R41  19.45,18.17 180 bottom
R42  1.45,29.45 90 bottom
R44  43.13,21.54 90 bottom
R45  39.25,21.54 90 bottom
R46  5.63,13.54 90 top
R47  7.51,13.54 90 top
R54  22.02,30.18 0 bottom
R61  16.11,32.25 180 bottom
R111  22.04,25.5 180 bottom
TP1  53.7,45.5 0 bottom
TP2  5.39,18.75 270 top
TP3  58.7,45.5 0 bottom
TP4  5.46,4.66 0 top
TP5  7.62,49.53 0 top
TP6  2.54,49.53 0 top
TP7  12.7,49.53 0 top
TP8  5.45,41.5 270 top
TP9  5.45,30.66 270 top
TP10  57.6,45.5 0 bottom
U1  45.72,27.94 0 top
U2  58.42,26.67 180 bottom
U3  14.8,14.89 90 top
U4  5.7,9.59 270 bottom
U5  19.05,35.15 270 top
U6  56.1,42.9 180 bottom
U7  41.91,10.16 0 bottom
U$1  not placed on the board
U$3  not placed on the board
U$6  [LT_LOGO_LARGE]  27.8,11.2 0 top
VSNSN1  26.67,28.8 270 top
VSNSN2  26.7,14.88 90 top
VSNSN3  26.68,12.56 0 top
VSNSN4  26.7,25.6 0 top
VSNSN11  26.67,34.52 270 top
VSNSN56  26.67,45.67 270 top
VSNSN57  26.67,43.81 270 top
VSNSN58  26.67,31.98 270 top
VSNSN59  26.67,30.07 270 top

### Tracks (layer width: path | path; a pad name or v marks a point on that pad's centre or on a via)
+12V  (via drill 0.25)
  Top 0.254: R11.2 R14.2 19.56,45.73 19.98,45.11 19.98,41.28 21.32,40.62 | U3.P$5 17.29,15.39 17.7,15.8 17.7,20.5 18.6,21.4 18.6,23.26 L2.1 | v21.4,18.2 21.5,18.3
  Bottom 0.254: R17.2 49.65,3.45 48.8,2.6 46.41,2.6 J1.VIN | R41.2 21.37,18.17 v21.4,18.2 | 11.25,1.85 R28.1
  Bottom 0.305: U7.P$1 42.86,10.12 42.85,10.13 40.95,10.13 40.95,8.87 U7.P$3 | C13.1 42.76,8.75
  Bottom 0.406: 42.76,8.75 U7.P$1 44.41,8.85 v44.45,8.89 | v19.4,1.8 18.9,1.3 12,1.3 11.25,1.85
  pour Top (no thermals): 20.17,36.12 20.41,36.12 20.41,41.08 27.4,41.08 27.4,35.48 20.17,35.48
  pour Top (no thermals): 27.35,35.48 20.14,35.48 20.14,25.3 17.9,25.3 17.9,0.9 18.52,0.93 18.58,0.92 27.4,0.98
  pour Top (no thermals): 24.13,0.98 47.39,1.01 47.39,8.86 44.7,11.5 33.9,11.5 27.4,17.7 24.13,17.73
  pour Top (no thermals): 21.5,25.3 21.5,20.8 17.9,20.8 17.9,25.3
ALERTB  (via drill 0.25)
  Top 0.254: U1.P$17 50.03,28.44 v50.8,28.47 | LED4.C 36.98,39.82 37.3,39.5 v39,39.5
  Route2 0.254: v38.1,45.62 v50.8,45.62 | v39,39.5 50.4,39.5 v50.8,39.1
  Route15 0.254: v50.8,28.47 v50.8,39.1 v50.8,45.62
  Bottom 0.254: v38.1,45.62 38.1,47.84 R2.1
ASEL0  (via drill 0.25)
  Top 0.254: U1.P$22 45.72,31.75 v46.99,33.02
  Route2 0.254: v52.07,33.02 v46.99,33.02
  Route15 0.254: JP1.2 52.07,17.78 v52.07,33.02
  Route15 0.406: JP1.3 JP1.2
ASEL1  (via drill 0.25)
  Top 0.254: U1.P$21 46.22,30.98 v46.99,31.75
  Route2 0.254: v57.15,31.75 v46.99,31.75
  Route15 0.254: JP2.2 58.42,16.51 57.15,17.78 v57.15,31.75
  Route15 0.406: JP2.3 JP2.2
AUX_VCC  (via drill 0.25)
  Route15 0.406: v60.9,39.7 60.9,44.4 61.9,45.4 J3.1
  Bottom 0.254: 59.3,30.51 C3.1
  Bottom 0.406: 59.3,30.51 59.3,32.8 57.65,34.45 R23.2 R25.2 57.65,38.85 58,39.2 60.4,39.2 v60.9,39.7 | U2.4 59.75,30 C3.1
AUXSCL  (via drill 0.25)
  Route2 0.254: v55.5,35.4 J3.11
  Route15 0.254: v55.5,25.7 v55.5,35.4
  Bottom 0.254: J3.11 R23.1
  Bottom 0.406: U2.1 55.52,25.72 v55.5,25.7
AUXSDA  (via drill 0.25)
  Route2 0.254: v54.6,37.3 60.5,37.3 61.4,36.4 63.5,36.4 J3.12
  Route15 0.254: v54.6,27.7 v54.6,37.3
  Bottom 0.254: J3.12 64.5,35.5 63.6,36.4 61.4,36.4 60.5,37.3 R25.1 | U2.3 54.68,27.62 v54.6,27.7
GND  (via drill 0.25)  (91 unrouted)
  Top 0.254: U1.P$24 44.72,28.94 U1.P$25 | Q1.S 17.86,42.51 17.42,42.95 15.26,42.95 v15.04,43.18 | U3.P$14 14.39,13.39 v14.2,13.5 | LED3.C 40.44,5.76 41.2,5 41.2,2.62 J1.GND1 | LED6.C v49.65,1.55 | LED5.C 33.1,38.7 v33.2,38.6
  Route2 0.254: v49.65,1.55 49,0.9 44.7,0.9 43.8,1.8 43.8,2.52 J1.GND2
  Bottom 0.254: v33.2,38.6 33.3,38.5
  other vias: 17.6,33.41 18.65,35.65 45.72,27.94 15.4,16.3 14.2,16.3 28.1,27.4 14.8,11.8 14.8,9.8 14.8,8.8 14.8,10.8 12.6,10.8 12.6,11.8 12.6,7.6 12.6,9.8 9.3,15.4 10.3,15.4 9.3,12.6 10.3,12.6 9.8,12 11.3,15.4 1.2,13.3 1.2,12.3 1.2,11.3 1.2,10.4 2.1,10.4 3.1,10.4 15.4,13.5 15.4,14.9 14.2,14.9 9.3,11.4 10.3,11.4 10.8,12 15,37.51 12,31.01 11,31.01 10,31.01 19.41,34.88
  pour Bottom (rank 3, no thermals): 65.85,51.57 65.77,40.07 68.3,37.34 68.3,5.79 65.67,3.21 65.67,0.94 0.9,0.94 0.9,52.3 65,52.4 65.33,52.07
  pour Top (rank 3, no thermals): 65.05,52.37 65.05,52.35 65.8,51.6 65.77,40.07 68.3,37.34 68.3,5.79 65.67,3.21 65.67,0.84 0.9,0.94 0.9,52.3 0.95,52.37
  pour Route2 (isolate 0.305, rank 3, no thermals): 65.85,51.57 65.77,40.07 68.3,37.34 68.3,5.79 65.67,3.21 65.67,0.94 0.9,0.94 0.9,52.4 0.95,52.37 65,52.4 65.33,52.07
  pour Route15 (isolate 0.305, rank 3, no thermals): 65.85,51.57 65.77,40.07 68.3,37.34 68.3,5.79 65.67,3.21 65.67,0.94 0.9,0.94 0.9,52.4 0.95,52.37 65,52.4 65.33,52.07
GPIO_0  (via drill 0.25)
  Top 0.254: U1.P$16 50.16,27.94 v50.8,27.38 | U5.14 21.39,35.02 21.6,34.8 21.6,34.2 21.27,33.87 v21.27,33.82
  Route2 0.254: v33.55,25.45 33.6,25.55 33.81,25.45 50.29,25.45 50.8,26.11 v50.8,27.38 | VSNSN11.1 25.97,33.82 v21.27,33.82
  Route15 0.254: v32.92,34.47 33.55,33.83 v33.55,25.45
  Bottom 0.254: R6.1 30.1,36.26 N4.G 28.57,35.54 28.6,35.13 | 28.6,35.13 29.26,34.47 v32.92,34.47 | VSNSN11.1 28.12,34.52 28.6,35.13
GPIO_1  (via drill 0.25)
  Top 0.254: U1.P$15 49.73,27.44 50.16,26.75 51.26,26.11 v51.26,25.02 | U3.P$11 12.81,14.89 v12.3,15.4
  Route2 0.254: VSNSN2.1 26.18,15.4 20.8,15.4 19.6,17 13.5,17 v12.3,15.4
  Route2 0.305: v31.75,16.51 50.95,16.51 v51.28,16.84
  Route15 0.305: v51.28,16.84 51.28,24.99 v51.26,25.02
  Bottom 0.254: 30.06,17.27 R5.1 29.89,17.13 N3.G 28.44,15.24 28.1,14.9 26.72,14.9 VSNSN2.1
  Bottom 0.305: R5.1 30.97,17.29 v31.75,16.51
GPIO_CFG  (via drill 0.25)
  Top 0.254: U1.P$20 46.86,30.48 v47.93,30.48
  Route2 0.254: v62.23,30.48 v47.93,30.48
  Route15 0.254: JP3.2 63.5,16.51 62.23,17.78 v62.23,30.48
INTVCC_LTC3604  (via drill 0.25)  (1 unrouted)
  Top 0.254: v20.4,37.63 19.81,37.23 U5.1 | U5.7 16.4,35.02 v16,35.31
  Top 0.305: U5.1 19.78,37.16 | U5.12 20.12,33.66 v20.4,33.45
  Route2 0.305: 20.39,33.44 20.39,33.86 20.11,34.22 17.02,34.22 v16,35.31
  Route15 0.305: v20.4,33.45 v20.4,37.63
  Bottom 0.254: 14.68,35.02 15.6,35.02 v16,35.31 | R54.1 22.87,30.33 22,31.2 22,32.8 21.6,33.2 20.65,33.2 v20.4,33.45 20.45,33.4
  Bottom 0.305: 14.68,35.02 C93.1
IOUT0  (via drill 0.25)
  Top 0.254: U1.P$14 48.93,26.94 v49.23,26.64
  Bottom 0.254: v49.23,26.64 49.53,26.34 R8.2
IOUT1  (via drill 0.25)
  Top 0.254: U1.P$13 48.16,26.44 v48.46,26.14
  Bottom 0.254: v48.46,26.14 48.49,24.36 47.62,23.52 R16.2
ISNSN_CH0  (via drill 0.25)
  Top 0.254: U1.P$4 42.19,27.94 v41.76,28.22
  Route2 0.254: v41.76,28.22 v29.18,28.22 | VSNSN56.1 15.72,45.67 v14.88,45.63
  Route15 0.254: v29.18,28.22 29.18,45.01 28.52,45.67 VSNSN56.1
  Bottom 0.254: 13.8,45.67 C12.1 13.84,45.63 v14.88,45.63
  Bottom 0.305: C12.1 R21.1
ISNSN_CH1  (via drill 0.25)
  Top 0.254: U1.P$8 44.66,25.6 44.2,25.6 43.8,25.2 43.8,22.9 v44.3,22.4
  Bottom 0.254: v44.3,22.4 42.94,22.4 R44.2
  Bottom 0.406: R45.1 41.06,20.69 C4.1 41.25,20.65 42.7,22.1 42.84,22.1 R44.2
ISNSP_CH0  (via drill 0.25)
  Top 0.254: U1.P$3 42.98,28.44 v42.32,28.91
  Route2 0.254: v42.32,28.91 32.79,28.88 v28.07,28.88
  Route15 0.254: v28.07,28.88 28.04,43.1 27.33,43.81 VSNSN57.1
  Bottom 0.254: R22.1 24.95,43.81 VSNSN57.1
  Bottom 0.305: 24.85,45.62 C16.2 24.85,43.92 R22.1
ISNSP_CH1  (via drill 0.25)  (1 unrouted)
  Top 0.254: U1.P$7 43.18,26.44 v42.95,26.11 42.95,24.55 v42.6,24.2
  Route2 0.254: v42.95,26.11 30.45,26.21 29.9,25.65 26.65,25.65 | v24.8,7.3 13.8,7.3 13,8.4 v4,8.4
  Route15 0.254: v24.8,7.3 24.8,24.5 VSNSN4.1
  Bottom 0.254: v4,8.4 U4.P$4
  Bottom 0.406: R45.2 39.25,23.65 39.8,24.2 41.6,24.2 | 41.6,24.2 v42.6,24.2 | C4.2 41.1,23.7 41.6,24.2
N$1  (via drill 0.25)
  Top 0.254: LED1.C v27.13,39.95
  Bottom 0.254: v27.13,39.95 27.13,37.56 N4.D
N$2  (via drill 0.25)
  Top 0.254: v30.1,42.8 28.04,42.8 LED1.A
  Bottom 0.254: R4.1 30.18,42.53 v30.1,42.8
N$3  (via drill 0.25)
  Top 0.254: v26.98,20.83 LED2.C
  Bottom 0.254: N3.D 26.98,18.43 26.95,18.47 v26.98,20.83
N$4  (via drill 0.25)
  Top 0.305: v27.89,23.27 LED2.A
  Bottom 0.305: R7.1 28.61,22.54 v27.89,23.27
N$5  (via drill 0.25)
  Top 0.254: R47.1 7.51,11.71 v7.5,11.6
  Bottom 0.254: U4.P$1 7.1,10.6 7.5,11 v7.5,11.6
N$6  (via drill 0.25)
  Top 0.254: LED3.A v36.16,5.76
  Bottom 0.254: v36.16,5.76 R10.1
N$7  (via drill 0.25)
  Top 0.254: LED4.A v38.08,42.31
  Bottom 0.254: v38.08,42.31 R9.1
N$8
  Bottom 0.254: R61.1 15.26,30.72 R27.2
N$9  (via drill 0.25)
  Top 0.254: v34.5,39 34.5,40.9 33.7,41.7 33.15,41.7 LED5.A
  Bottom 0.254: R12.1 33.6,39.9 v34.5,39
N$10
  Bottom 0.254: P2.D 33.4,41.85 R12.2
N$11  (via drill 0.25)
  Top 0.254: LED6.A 48.15,4.55 v48.1,4.5
  Bottom 0.254: v48.1,4.5 48.1,6.85 R17.1
N$12
  Bottom 0.254: U4.P$9 6.2,9.09 U4.P$3
  Bottom 0.406: C7.2 5.7,8.35 U4.P$9 6,9.89 6,10.1 6.4,10.5 6.4,11 6.6,11.2 R29.2
N$13  (via drill 0.25)
  Route15 0.406: v7.7,1.2 8.4,1.9 8.4,6.3 7.9,6.8 v7.7,6.8
  Bottom 0.254: C7.1 7.1,7.6 7.8,8.4 7.8,9.6 U4.P$2
  Bottom 0.406: R28.2 8.4,1.9 v7.7,1.2 | v7.7,6.8 7.45,6.8 C7.1
N$14
  Bottom 0.406: C8.1 R31.1
N$15  (via drill 0.25)
  other vias: 15.4,25.5 16,24.8 12.9,24.1 16.6,24.1 15.4,24.1 14.1,24.1 12.9,25.5 14.8,24.8 14.2,25.5 16.6,25.5 13.5,24.8
  pour Bottom (isolate 0.305, no thermals): 16.8,21.6 16.8,25.8 11.2,25.8 8.4,23.6 8.4,21.6
  pour Top (isolate 0.305, no thermals): 16.8,23.9 16.8,26.4 16.5,27.4 13.1,27.4 12.7,26.4 12.7,23.9
N$16
  Bottom 0.406: R3.1 66.02,18.58 JP3.1
N$18  (via drill 0.25)
  other vias: 16.6,17.7 15.7,17.7 13.9,17.7 12.9,17.7 12.9,20.3 14.8,17.7 16.7,20.3
  pour Top (isolate 0.254, no thermals): 16.9,15.8 16.9,20.4 12.7,20.4 12.7,15.8
  pour Bottom (isolate 0.305, no thermals): 16.9,17.6 16.9,19.3 18.9,19.3 18.9,20.4 12.8,20.4 12.8,17.6
N$19  (1 unrouted)
  Top 0.254: 16.53,44.07 15.8,44.8
  Top 0.305: P1.A 15.8,44.8
N$20
  Top 0.254: P1.C 9.13,43.77 13.07,43.77 13.58,43.26 13.62,43.26 13.62,42.65 14.15,42.01 Q1.D
N$21  (via drill 0.25)
  Top 0.254: U3.P$4 16.91,14.89 v17.3,14.8
  Bottom 0.254: R41.1 17.97,18.17 17.5,17.7 17.5,15 v17.3,14.8
N$22  (via drill 0.25)
  Top 0.254: U3.P$12 12.21,14.39 v12.23,14.37
  Route15 0.254: v12.23,14.37 12.2,14.4 12.1,14.4 11.6,13.9 11.6,8.2 11.1,7.7 10.8,7.7 10.3,7.2 v10.3,6.6
  Bottom 0.254: v10.3,6.6 10.3,6.03 R36.1
N$23  (via drill 0.25)  (1 unrouted)
  Top 0.254: U3.P$13 12.69,13.89 12.2,13.5
  Route15 0.254: v12.25,13.5 12.9,13.5 13.4,13.1 13.4,7.1 12.9,6.6 v11.1,6.6
  Bottom 0.254: C20.2 11.05,3.65 11.9,4.5 11.9,6.3 11.6,6.6 v11.1,6.6
N$25
  Top 0.254: Q1.G 19.01,41.51 19.11,41.41 | U5.2 19.28,41.23 19.11,41.41 | R11.1 18.57,44.03 19.3,43.3 19.3,41.6 19.11,41.41
N$26
  Bottom 0.254: U6.8 58.05,43.65 58.8,44.4 58.8,45.4 TP3.P$1
N$27  (via drill 0.25)
  Top 0.254: v7.5,25.5 7.3,25.5 6.9,25.1 6.9,23.4 7.5,22.8 8.2,22.8 R35.2
  Top 0.406: v7.4,15.4 7.4,14.5 R47.2
  Route2 0.254: v7.4,15.4 7.7,15.4 8.6,16.3 8.6,24.4 v7.5,25.5
  Bottom 0.406: R29.1 6.6,14.7 v7.4,15.4
  pour Top (rank 2, no thermals): 12,24.9 7.7,24.9 7.7,20.9 8.5,20.4 8.5,16.2 12,16.2
N$28  (via drill 0.25)
  Top 0.254: P3.A 9.58,27.72 9.1,28.2 7.2,28.2 6.9,27.9 v2.6,27.9
  Bottom 0.254: v2.6,27.9 2.55,27.9 R42.1
N$29
  Bottom 0.254: U6.7 57.55,45.45 TP10.P$1
N$30
  Bottom 0.254: U6.5 54.15,43.65 53.6,44.2 53.6,45.4 TP1.P$1
N$31
  Bottom 0.305: C22.2 20.4,14.43 R38.2
N$32  (via drill 0.25)
  Top 0.254: U3.P$2 v17.29,13.89
  Bottom 0.254: v17.29,13.89 17.96,13.89 R38.1 18.6,16.29 C21.2
N$33  (via drill 0.25)
  Top 0.254: R46.1 5.63,11.67 v5.7,11.6
  Bottom 0.254: v5.7,11.6 5.7,10.8 5.5,10.6 4.81,10.6 U4.P$6
N$70
  Top 0.254: U5.6 16.73,35.52 16.36,35.89 C31.2
N$78  (via drill 0.25)
  Top 0.305: U5.10 18.78,32.88 v18.3,32.48
  Route2 0.254: v20.2,31.2 20.2,31.4 19.9,31.7 19.18,31.7 v18.3,32.48
  Bottom 0.254: R54.2 21.17,30.23 v20.2,31.2
REF  (via drill 0.25)
  Top 0.254: U1.P$23 45.22,31.36 v44.98,31.6
  Bottom 0.254: v44.98,31.6 45.21,31.83 C1.1
SCL  (via drill 0.25)
  Top 0.254: U1.P$18 49.26,28.94 v49.84,29.18
  Route2 0.254: TP7.TP1 13.97,50.8 J1.SCL 19.43,50.42 20.32,49.53 41.91,49.53 v44.45,46.99 v49.84,46.99 | v35,43.1 49.23,43.1 v49.84,42.4
  Route15 0.254: v49.84,46.99 v49.84,42.4 v49.84,29.18
  Bottom 0.254: v44.45,46.99 44.39,46.99 R0.1 | v35,43.1 34.55,43.55 P2.G | U6.4 50.59,43.15 v49.84,42.4 50.75,41.48 R32.1
SCL_DONGLE  (via drill 0.25)
  Route2 0.254: v53.5,42.3 53.6,42.4 63.5,42.4 J3.4
  Bottom 0.254: U6.3 53.85,42.65 v53.5,42.3 52.6,41.4 R32.2
SDA  (via drill 0.25)
  Top 0.254: U1.P$19 48.49,29.44 48.9,29.84 48.9,29.89 v48.9,29.8
  Route2 0.254: TP6.TP1 2.54,50.8 3.81,52.07 21.59,52.07 21.97,51.69 J1.SDA 22.01,50.76 22.01,51.22 22.86,52.07 43.18,52.07 44.45,50.8 44.45,49.3 v48.92,49.3 v57.7,49.3
  Route15 0.254: v48.9,29.8 48.9,49.28 v48.92,49.3 | v59,43.5 59,47.6 | v57.7,49.3 59,48 59,47.8 59,47.6 | v60,47.6 59,47.6
  Bottom 0.254: R1.1 48.04,48.08 v48.92,49.3 | U6.9 58.65,43.15 v59,43.5 | R33.1 v60,47.6
SDA_DONGLE  (via drill 0.25)
  Route2 0.254: v59.7,43.1 59.7,43.9 60.1,44.4 63.5,44.4 J3.2
  Bottom 0.254: U6.10 59.25,42.65 v59.7,43.1 60,43.4 R33.2
SW1
  pour Top (no thermals): 18.8,36.4 18.8,41.05 13.21,41.05 13.21,38.2 17.02,38.23 18.26,37.13 18.26,36.4
V1  (via drill 0.25)
  Top 0.254: L7.2 10.79,39.29 | U5.8 15.88,34.52 15.3,35.1 15.3,36.4 14.8,36.9 12.26,36.9 v12.2,36.85
  Route2 0.254: v21.84,44.37 15.19,44.37 13.92,43.1 10.81,43.1 10.1,42.4 10.1,39.9 9.65,39.55 v9.4,39.55
  Bottom 0.254: R22.2 22.07,43.84 v21.84,44.37
  other vias: 9.6,41.15 10.8,41.15 12,41.15 12.2,40.05 12.2,39.05 12.2,38.05
  pour Top (no thermals): 12.73,42.19 12.73,34.83 9.19,34.83 9.19,42.19
  pour Bottom (no thermals): 9.2,36.3 12.7,36.3 12.7,42.2 9.2,42.2
V3V3_DONGLE
  Bottom 0.254: U6.11 61.75,42.15 J3.5
V5REF  (via drill 0.25)
  Top 0.254: U1.P$5 v41.48,27.44
  Route2 0.254: v34.8,27.43 34.81,27.43 v41.48,27.44 | v22,11.7 22.8,10.9 33,10.9 33.81,11.71 33.81,11.72
  Route2 0.305: 33.81,11.72 v33.81,12.72
  Route15 0.254: v34.8,27.43 34.29,26.92 34.29,13.21 v33.81,12.72
  Bottom 0.254: R18.2 v33.82,12.74 v33.81,12.72 | R26.2 18.67,11.37 19.1,11.8 21.9,11.8 v22,11.7
  Bottom 0.305: C5.1 42.76,11.57 U7.P$5
  Bottom 0.406: R18.2 35.2,13.72 35.81,14.33 41.77,14.33 C5.1
VDD  (via drill 0.25)  (5 unrouted)
  Top 0.254: v45.72,23.98 U1.P$10 U1.P$9 45.22,24.9 v44.7,23.98
  Route2 0.254: v31.34,40.84 v38.2,40.84 40.57,40.84 v40.64,40.91 | 40.75,46.3 v45.1,46.3 | v53.9,40.6 40.8,40.6 40.6,40.9 | 40.75,46.3 v40.64,46.41 | 40.75,46.3 33.3,46.3 v32.3,44.9
  Route2 0.406: v32.3,18.9 32.7,18.5
  Route2 0.61: JP2.1 JP1.1 53.3,18.52 v38.73,18.52 | 32.7,18.5 38.72,18.5
  Route15 0.254: 40.64,23.32 39.85,23.32 39.8,23.37
  Route15 0.61: v44.7,23.98 44.45,23.6 44.32,23.37 39.8,23.37 39.55,23.37 38.73,22.66 v38.73,18.52 v38.73,4.2 J1.5V | v40.64,46.41 v40.64,40.91 40.64,23.32
  Bottom 0.254: v45.72,23.98 C2.1 | R6.2 30.23,39.89 | 30.23,39.89 R4.2 | 30.23,39.89 31.36,40.84 | 29.96,20.84 R7.2 | 39.97,48.01 R2.2 39.94,47.1 v40.64,46.41 41.67,47.44 R0.2 | R10.2 31.38,4.72 31.8,4.3 38.63,4.3 v38.73,4.2 | R9.2 37.35,39.95 38.2,40.8 v38.2,40.84 | JP2.1 61.41,20.28 R3.2 67.48,20.28 68.3,21.1 68.3,29.6 67.4,30.5 66.82,30.5 J1.5V1 | v45.1,46.3 45.6,46.7 45.6,47.97 | U6.12 57.5,41.6 57.5,41.1 57,40.7 55.2,40.7 54.65,41.25 U6.1 54.65,41.35 v53.9,40.6 | P2.S 32.9,44.3 v32.3,44.9
  Bottom 0.305: R5.2 30.11,19.05
  Bottom 0.406: R7.2 30,20.84 30,18.9 v32.3,18.9
VFB0  (via drill 0.25)
  Top 0.254: 19.7,32.28 v19.68,32.3
  Top 0.305: U5.11 19.28,32.85 v19.68,32.3
  Route15 0.254: v19.68,32.3 18.1,31.1 18.02,31.02 v18.02,30.05
  Bottom 0.254: 18.78,29.25 18.84,29.2 18.93,29.2 C35.2 18.13,30.05 v18.02,30.05 | R24.2 17.82,30.05 v18.02,30.05 | R27.1 17.37,30.71 v18.02,30.05
  Bottom 0.305: v19.68,32.3 20.99,32.3 R13.1
VFB1  (via drill 0.25)
  Top 0.254: U3.P$1 v17.35,13.02
  Route2 0.254: 17.32,13.02 v17.35,13.02 17.38,13.02 17.9,12.5 26.64,12.52 VSNSN3.1 26.85,12.53 32.57,12.53 32.9,12.2 v32.9,11.9 v32.91,11.89
  Route15 0.254: 26.7,12.54 VSNSN3.1 | v21.3,6.2 18,6.2 17.4,6.8 17.4,12.97 v17.35,13.02
  Bottom 0.254: v32.91,11.89 33.39,11.9 33.86,11.9 34.29,11.47 34.29,7.62 34.68,7.23 R20.1 | R30.2 20.45,7.05
  Bottom 0.406: 20.45,7.05 v21.3,6.2
VOUT0  (via drill 0.25)
  Top 0.254: U1.P$11 46.22,24.9 v46.99,24.13
  Route2 0.254: v46.99,24.13 46.18,24.94 38.41,24.94 v38.1,24.73 | v38.1,31.98 VSNSN58.1
  Route15 0.254: v38.1,24.73 v38.1,31.98
  Bottom 0.254: R13.2 22.82,31.98 VSNSN58.1
VOUT1  (via drill 0.25)
  Top 0.254: U1.P$12 47.13,25.54 v47.73,24.84
  Route2 0.254: v46.99,12.7 37.39,12.7 37.31,12.62 v37.31,11.73
  Route15 0.254: v47.73,24.84 47.73,13.44 v46.99,12.7
  Bottom 0.254: R20.2 R18.1 36.62,11.04 v37.31,11.73
VOUT_CH0  (via drill 0.25)
  Route2 0.254: TP8.TP 5.5,41.45 5.5,34.8 6.3,34 15.3,34 19.3,30.2 v20,30.2
  Route15 0.254: v20,25.5 v20,30.2
  Bottom 0.254: R111.1 20.8,25.5 v20,25.5 | R61.2 16.96,32.16 | 17,32.2 R61.2 | R61.2 16.96,32.54 | 6.93,43.1 6.93,42.99 TP8.TP | v20,30.2 19.58,30.2 C35.1 17.53,32.25 R61.2 | 11.21,43.1 10.91,42.8 9.6,42.8 8.8,42 8.8,39.1 7.52,37.82 R19.2
  Bottom 0.305: R21.2 11.21,43.1
  pour Top (isolate 0.254, rank 2, no thermals): 8.84,42.24 8.84,34.84 0.92,34.84 0.92,44.14 7.1,44.1 7.16,44.04
  pour Bottom (no thermals): 2.54,44.45 2.54,36.43 8.2,36.4 8.23,36.83 8.23,44.45
VOUT_CH1  (via drill 0.25)  (1 unrouted)
  Top 0.254: R46.2 5.6,14.42 | v6.9,21.3 6.9,22.3 6.3,22.9 R35.1
  Top 0.406: P3.C 8.08,26.98 5.5,25.1 R35.1 | 5.6,14.42 v5.6,15.4
  Route2 0.254: 5.5,18.7 6.6,17.8 6.6,10.1 7.8,9.1 13.6,9.1 14.4,8 v19.5,8
  Route15 0.254: v5.6,15.4 5.6,15.8 5.9,16.1 7.2,16.1 7.7,16.6 7.7,20.5 v6.9,21.3
  Bottom 0.406: R34.1 18.67,8.83 v19.5,8 18.68,7.18 R30.1
  pour Top (no thermals): 1,14.1 4.4,14.1 4.4,16.2 7.7,16.2 7.7,19.7 6.1,21 6.1,26.4 1,26.4
VSNSN_CH0  (via drill 0.25)
  Top 0.254: U1.P$2 43.42,28.94 v42.7,29.67
  Route2 0.254: v42.7,29.67 27.53,29.67 VSNSN1.1
  Bottom 0.254: VSNSN1.1 23.07,28.8 R15.2
VSNSN_CH1  (via drill 0.25)
  Top 0.254: U1.P$6 42.18,26.94 v42.01,26.77
  Route2 0.254: v42.01,26.77 v29.21,26.77 | v21.52,9.97 v28.42,9.97
  Route15 0.254: v28.42,9.97 29.21,10.76 v29.21,26.77
  Bottom 0.406: v21.52,9.97 20.63,9.97 | 20.63,9.97 20.4,10.2 20.4,10.84 R26.1 | 20.63,9.97 20.63,9.93 20.4,9.7 20.4,9.07 R34.2
VSNSP_CH0  (via drill 0.25)
  Top 0.254: U1.P$1 43.82,30.04 v43.16,30.71
  Route2 0.254: v43.16,30.71 27.3,30.71 VSNSN59.1
  Route15 0.254: VSNSN59.1 24.87,30.07 23.9,29.1 23.9,26.23 v23.89,26.22
  Bottom 0.254: C99.2 22.89,27 23.11,27 v23.89,26.22 23.17,25.5 R111.2

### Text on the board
tPlace: - | +
tNames: SDA | GND | SCL | DC1613 CONNECTOR | VOUT_CH0 | PGOOD0 | GPIO_0 | SCL | ALERT | GND | LTC2970 | PGOOD1 | VOUT_CH1 | GPIO_1 | ASEL0 | ASEL1 | GPIO_CFG | DC2467A | HI | HI | LTC2970 WITH +5V and -5V / REGULATED SUPPLIES | Z | LO | LO | www.linear.com (408) 432-1900 | GND | VDD_5V | VDD_12V
bNames: ISNSN_0 | ISNSP_0 | GPIO0 | VOUT0 | VSNSP0 | VSNSN0 | ISNSP_CH1 | GPIO1 | VFB1 | 2
bAssembly: BOTTOM ASSEMBLY DRAWING
d_TopAssembly: NOTES: UNLESS OTHERWISE SPECIFIED | 1. WORKMANSHIP SHALL BE IN ACCORDANCE WITH IPC-A-610 | 6. INSTALL J1 HEADERS WITH LONG PINS POINTED OUT / OF THE BOTTOM OF THE BOARD (DOWN). | 2. PARTS TO OMIT WILL BE SPECIFIED ON THE BILL OF MATERIALS. / MASK THE SOLDER STENCIL WHERE PARTS ARE OMITTED. | 7. INSTALL SHUNTS AS SHOWN. | 3. DEPANELIZE BOARDS AFTER ASSEMBLY AND ROUTE OUT / THE BREAKOUT TABS ON ALL EDGES. | 8. MIND THE POLARITY OF C91 AND ALL LEDS | 4. ASSY PROCESS WILL INCLUDE: REFLOW SOLDER TOP SIDE SMD. | 5. DO NOT APPLY ANY KIND OF ASSEMBLY STAMP OR QA STAMP / ON ANY BOARD | TOP ASSEMBLY DRAWING
d_FabDrawing: NOTES: UNLESS OTHERWISE SPECIFIED | 1. WORKMANSHIP SHALL BE IN ACCORDANCE WITH IPC-A-600 | 5. DRILL: PLATE THRU ALL HOLES WITH COPPER, 0.001" THICK MIN. / ALL HOLES DRILLED +/-0.003" WITH RESPECT TO CTR. OF DRILLED PAD. / ALL HOLES FINISHED SIZE AFTER PLATING. | 2. MATERIAL: EPOXY FIBERGLASS, NEMA GRADE FR-4 / 4-LAYER BOARD, 2 OZ CU ON OUTER LAYERS / 1 OZ CU ON INNER LAYERS / FLAMMABILITY RATING: 94 V-2 MINIMUM | 6. DROP ALL UNUSED PADS ON INNER LAYERS. | 7. DO NOT ALTER ARTWORK e.g. TO ADD LOGO OR DATE CODE | 8. PCBs ARE TO BE RoHS COMPLIANT. | 3. SIZE: CUT TO DIMENSIONS AND TOLERANCES SHOWN. / 0.00 ARE PRIMARY DATUMS | 4. FINISH: SMOBC USING LPI BOTH SIDES, COLOR BLACK / ENIG FINISH. LEAD FREE SOLDER FOR PROTOTYPES / HIGH DEFINITION WHITE SILKSCREEN. | 53.3mm | 0.00 | 0.00 | 69.2mm | DRILL TABLE | FAB DRAWING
